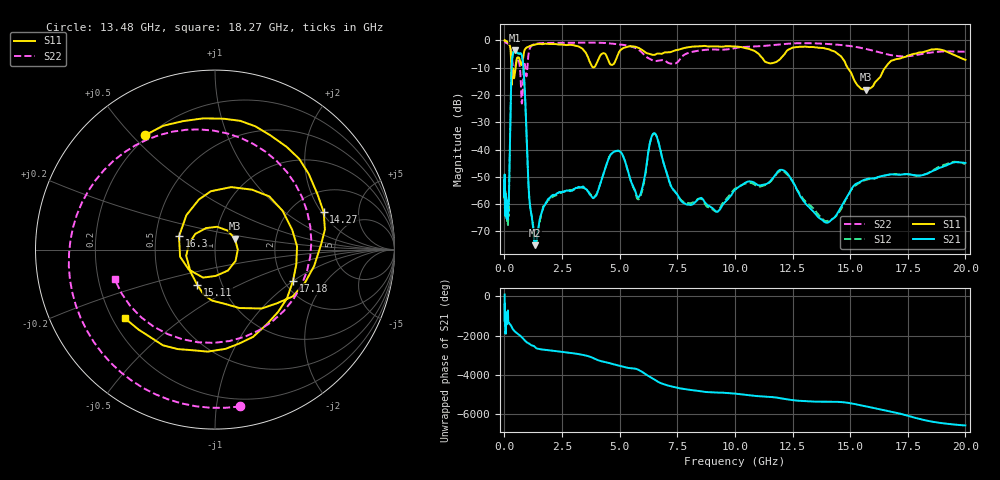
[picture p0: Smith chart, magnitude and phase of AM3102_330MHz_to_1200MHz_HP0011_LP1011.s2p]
! Date/Time: Tue, Sep 11, 2018 5:12 PM
! Network Analyzer: Agilent Technologies E8362B Rev: A.07.50.63
! Sweep from 0.010 to 20.000 GHz, 1601 Points, Sweep Type: LOG
! Power Supply: 4.949 V, 0.001 A
# Hz S DB R 50
!freq MagS11 AngS11 MagS21 AngS21 MagS12 AngS12 MagS22 AngS22
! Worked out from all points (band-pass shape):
!   1601 points, 10 MHz to 20 GHz, reference 50 ohm
!   highest |S21| = -3.60 dB at 449.3 MHz (marker M1); lowest = -75.1 dB at 1.334 GHz (marker M2)
!   |S21| within 3 dB of the highest: 338.2 MHz to 784.8 MHz (446.6 MHz wide, 79.5 % of centre)
!   lowest |S11| = -18.0 dB at 15.7 GHz (marker M3), VSWR 1.29, Z = 61.9 + j7.61 ohm
!   |S11| at or under -10 dB: 298.9 MHz to 488.2 MHz (189.3 MHz wide, 48.1 % of centre); 14.89 GHz to 16.52 GHz (1.625 GHz wide, 10.3 % of centre)
!   |S22| runs from -23.1 to -0.3 dB; largest |S21 - S12| = 0.012
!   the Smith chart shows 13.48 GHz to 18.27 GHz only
!   S11 on the Smith chart (normalised r, x): 13.48 GHz: 0.19, +0.55; 14.27 GHz: 2.96, +2.10; 15.11 GHz: 0.76, -0.31; 16.3 GHz: 0.66, +0.10; 17.18 GHz: 2.23, -1.00; 18.27 GHz: 0.25, -0.32
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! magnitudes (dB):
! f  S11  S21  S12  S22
! 10 MHz  0.0  -51.3  -54.6  -0.3
! 35.55 MHz  0.0  -62.8  -63.4  -0.5
! 126.4 MHz  -0.4  -62.7  -64.8  -1.1
! 190.2 MHz  -1.1  -58.3  -60.7  -1.4
! 313.2 MHz  -15.5  -9.9  -9.9  -5.3
! 447.2 MHz  -12.4  -3.6  -3.7  -11.0
! 449.3 MHz  -12.3  -3.6  -3.6  -10.9
! 802.2 MHz  -7.1  -7.8  -7.8  -16.1
! 1.334 GHz  -1.5  -75.1  -74.5  -1.3
! 1.59 GHz  -1.3  -64.0  -64.0  -1.0
! 4.832 GHz  -7.2  -40.5  -40.6  -1.3
! 5.652 GHz  -2.3  -54.7  -54.9  -2.6
! 6.518 GHz  -5.2  -34.0  -34.1  -7.5
! 7.845 GHz  -2.7  -59.8  -59.4  -5.1
! 13.48 GHz  -2.5  -63.5  -62.2  -1.1
! 14.27 GHz  -3.9  -65.2  -65.2  -1.4
! 15.11 GHz  -13.2  -53.7  -54.1  -2.2
! 15.7 GHz  -18.0  -50.9  -51.1  -3.1
! 16.3 GHz  -13.4  -49.8  -49.9  -4.4
! 17.18 GHz  -6.6  -49.2  -49.1  -5.8
! 18.27 GHz  -4.0  -49.0  -49.0  -4.7
! 20 GHz  -7.1  -44.9  -45.3  -4.1
